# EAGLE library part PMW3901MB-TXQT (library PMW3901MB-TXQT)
PMW3901MB-TXQT Source: Datasheet
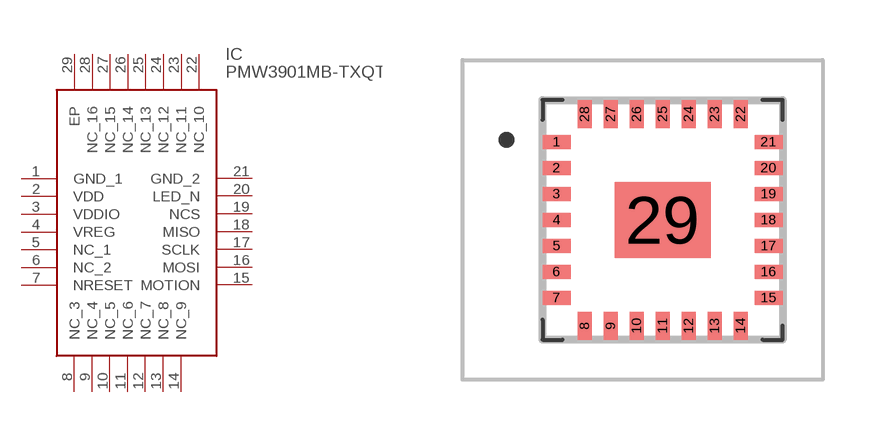
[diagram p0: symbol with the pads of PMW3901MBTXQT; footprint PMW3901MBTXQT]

Designator prefix IC

## PMW3901MB-TXQT (Arrow_Part_Number: PMW3901MB-TXQT; Description: PMW3901MB-TXQT; Height: 2.36mm; Manufacturer_Name: PixArt Imaging Inc.; Manufacturer_Part_Number: PMW3901MB-TXQT)  [PMW3901MBTXQT]
1  GND_1
2  VDD
3  VDDIO
4  VREG
5  NC_1
6  NC_2
7  NRESET
8  NC_3
9  NC_4
10  NC_5
11  NC_6
12  NC_7
13  NC_8
14  NC_9
15  MOTION
16  MOSI
17  SCLK
18  MISO
19  NCS
20  LED_N
21  GND_2
22  NC_10
23  NC_11
24  NC_12
25  NC_13
26  NC_14
27  NC_15
28  NC_16
29  EP

## Footprint PMW3901MBTXQT (pad centres in mm)
PMW3901MB-TXQT-2
smd 0.7 x 0.35: 1 -2.65,1.95; 2 -2.65,1.3; 3 -2.65,0.65; 4 -2.65,0; 5 -2.65,-0.65; 6 -2.65,-1.3; 7 -2.65,-1.95; 15 2.65,-1.95; 16 2.65,-1.3; 17 2.65,-0.65; 18 2.65,0; 19 2.65,0.65; 20 2.65,1.3; 21 2.65,1.95
smd 0.35 x 0.7: 8 -1.95,-2.65; 9 -1.3,-2.65; 10 -0.65,-2.65; 11 0,-2.65; 12 0.65,-2.65; 13 1.3,-2.65; 14 1.95,-2.65; 22 1.95,2.65; 23 1.3,2.65; 24 0.65,2.65; 25 0,2.65; 26 -0.65,2.65; 27 -1.3,2.65; 28 -1.95,2.65
smd 2.4 x 1.9: 29 0,0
